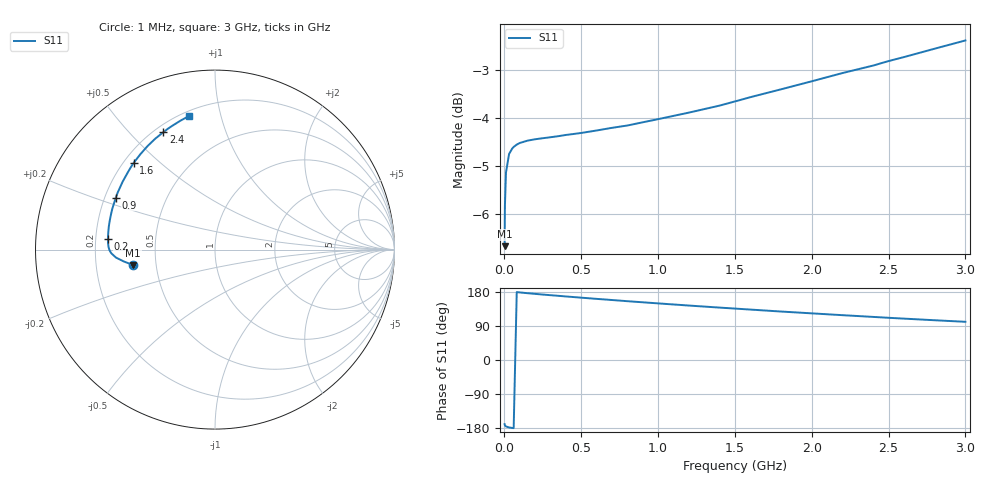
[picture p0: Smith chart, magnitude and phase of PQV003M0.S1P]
! SIEMENS Small Signal Semiconductors
! BAR64-04
! Si PIN Diode in SOT23 (2 diodes in series, pin 3 open)
! IF = 3 mA
! S-Parameters:  July  1992
# GHz  S  MA  R  50
!  f  S11
! GHz  MAG  ANG
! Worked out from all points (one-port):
!   33 points, 1 MHz to 3 GHz, reference 50 ohm
!   lowest |S11| = -6.7 dB at 1 MHz (marker M1), VSWR 2.73, Z = 18.4 - j4.05 ohm
!   |S11| at or under -10 dB: nowhere
!   S11 on the Smith chart (normalised r, x): 1 MHz: 0.37, -0.08; 200 MHz: 0.25, +0.05; 900 MHz: 0.24, +0.23; 1.6 GHz: 0.24, +0.41; 2.4 GHz: 0.23, +0.63; 3 GHz: 0.23, +0.80
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0.001  0.464 -169.3
0.003  0.5111 -172.5
0.01  0.5535 -175.4
0.03  0.5784 -178.0
0.05  0.5859 -179.3
0.08  0.5916 179.2
0.1  0.5939 178.3
0.15  0.5972 176.3
0.2  0.5992 174.5
0.25  0.6007 172.7
0.4  0.6054 167.7
0.5  0.6083 164.5
0.6  0.6119 161.3
0.7  0.6158 158.3
0.8  0.6192 155.2
0.9  0.624 152.3
1  0.6287 149.4
1.2  0.6386 143.7
1.5  0.6559 135.7
1.6  0.6626 133.1
1.8  0.6752 127.9
2  0.6883 123.1
2.2  0.702 118.3
2.4  0.7147 113.7
2.5  0.7224 111.4
2.6  0.7293 109.2
2.8  0.7441 104.9
3  0.7589 100.8
